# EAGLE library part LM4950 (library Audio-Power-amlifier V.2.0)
LM4950 Boomer ™ Audio Power Amplifier Series 7.5W Mono-BTL or 3.1W Stereo Audio Power Amplifier
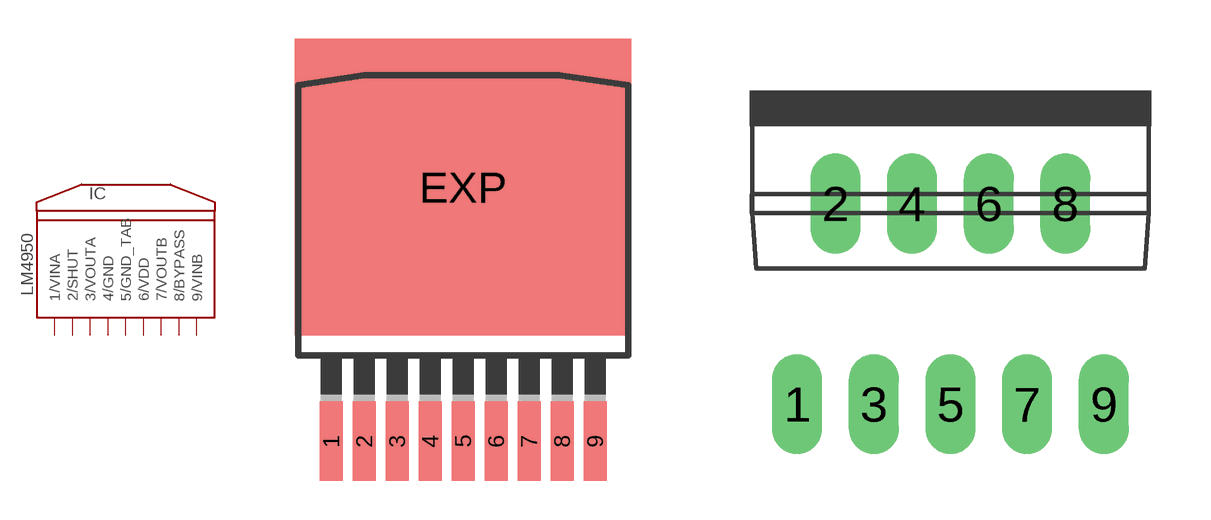
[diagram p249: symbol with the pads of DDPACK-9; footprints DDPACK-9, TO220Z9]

Designator prefix IC

## LM4950  [DDPACK-9]
1  1/VINA  in
2  2/SHUT
3  3/VOUTA  out
4  4/GND  pwr
5  5/GND_TAB  pwr
6  6/VDD  pwr
7  7/VOUTB  out
8  8/BYPASS
9  9/VINB  in

## LM4950TO220-9  [TO220Z9]
Pads as for DDPACK-9

## Footprint DDPACK-9 (pad centres in mm)
DDPAK-9
smd 0.889 x 3.048: 1 -5.08,-8.255; 2 -3.81,-8.255; 3 -2.54,-8.255; 4 -1.27,-8.255; 5 0,-8.255; 6 1.27,-8.255; 7 2.54,-8.255; 8 3.81,-8.255; 9 5.08,-8.255
smd 12.954 x 11.43: EXP 0,1.524

## Footprint TO220Z9 (pad centres in mm)
9-lead single in-line (TO220Z9) plastic power package
drill 0.5 pad 1.27 long: 1 -3.88,-5.08; 2 -2.91,0; 3 -1.94,-5.08; 4 -0.97,0; 5 0,-5.08; 6 0.97,0; 7 1.94,-5.08; 8 2.91,0; 9 3.88,-5.08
